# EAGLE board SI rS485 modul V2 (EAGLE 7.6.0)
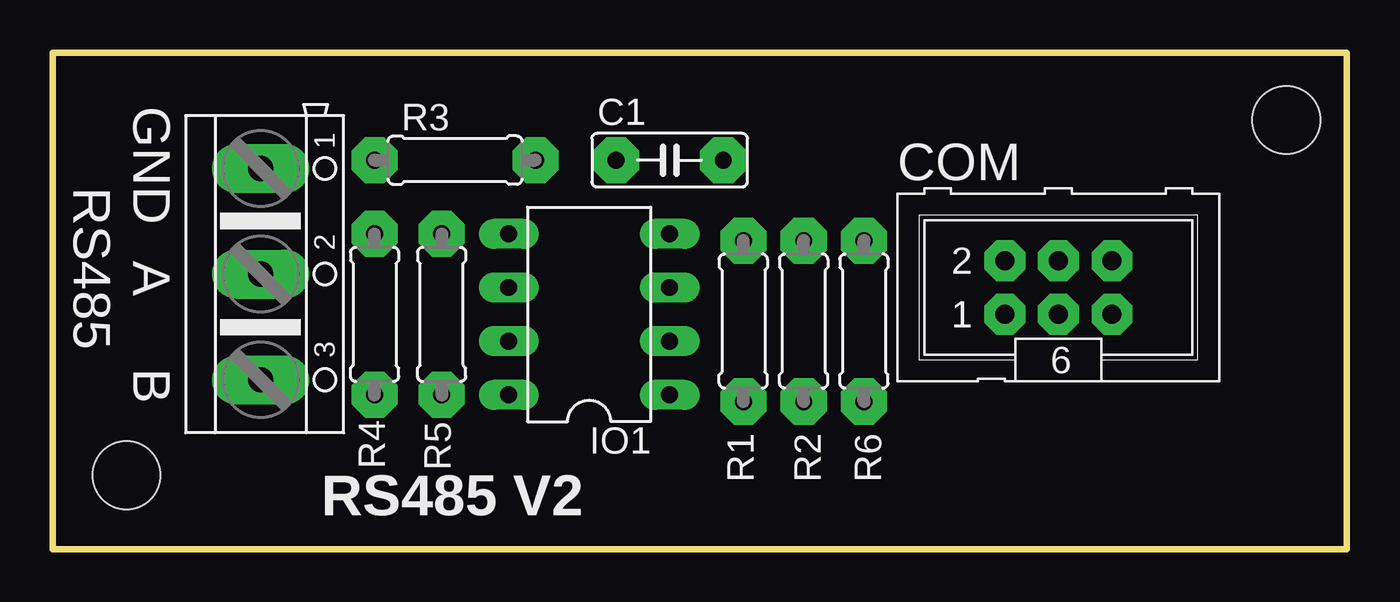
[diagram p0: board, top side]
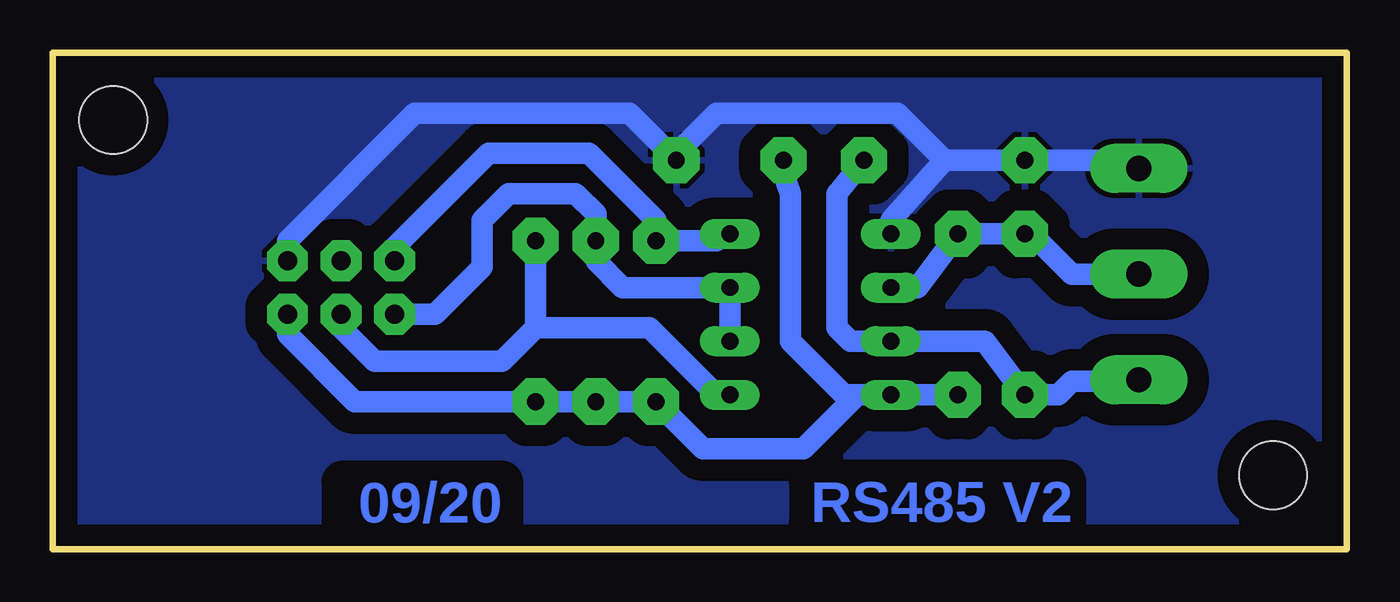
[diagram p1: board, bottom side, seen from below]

Size 61.28 x 23.5 mm. Coordinates in mm from the lower left corner, seen from the top.
Outline: 0,23.5 61.28,23.5 61.28,0 0,0 0,23.5
Copper layers (1*16): Top 0.035mm / dielectric 1.5mm / Bottom 0.035mm
Design rules "default": minimum track width 10mil, minimum drill 24mil, track to track 8mil, track to pad 8mil, pad to pad 8mil, via to via 8mil, smd to smd 8mil, copper to edge 40mil, drill to drill 8mil, minimum pad ring 10mil, minimum via ring 8mil, stop-mask expansion 4mil, vias tented up to drill 0mil, thermal gap 10mil
Holes 3.2 mm at 58.42,20.32 3.49,3.49

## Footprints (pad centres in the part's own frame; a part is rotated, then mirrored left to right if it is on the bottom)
C050-025X075 = drill 0.8 pad 2.184 octagon: 1 -2.54,0; 2 2.54,0
ML6 = drill 0.9 pad 1.93 octagon: 1 -2.54,-1.27; 2 -2.54,1.27; 3 0,-1.27; 4 0,1.27; 5 2.54,-1.27; 6 2.54,1.27
DIL08 = drill 0.8 pad 1.422 long: 1 -3.81,-3.81; 2 -1.27,-3.81; 3 1.27,-3.81; 4 3.81,-3.81; 5 3.81,3.81; 6 1.27,3.81; 7 -1.27,3.81; 8 -3.81,3.81
0207/7 = drill 0.8 pad 2.184 octagon: 1 -3.81,0; 2 3.81,0
AK500/3 = drill 1.2 pad 2.311 long: 1 -5.004,0; 2 0,0; 3 5.004,0

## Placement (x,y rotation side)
C1  100n  [C050-025X075]  29.21,18.41 0 top
COM  [ML6]  47.62,12.38 0 top
IO1  MAX485  [DIL08]  25.4,11.11 90 top
R1  10k  [0207/7]  32.7,10.79 90 top
R2  10k  [0207/7]  35.56,10.79 90 top
R3  20k  [0207/7]  19.05,18.41 0 top
R4  120  [0207/7]  15.24,11.11 90 top
R5  20k  [0207/7]  18.41,11.11 270 top
R6  10k  [0207/7]  38.42,10.79 90 top
RS485  [AK500/3]  9.84,13.02 270 top

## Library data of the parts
C1 COM IO1 R1-R6 RS485 = 11moje

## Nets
GND: C1.2 COM.6 IO1.5 R3.1 RS485.1
S$1: C1.1 COM.5 IO1.8 R1.1 R2.1 R5.2 R6.1
S$5: COM.1 IO1.2 IO1.3 R2.2
S$7: IO1.6 R4.2 R5.1 RS485.2
S$10: IO1.7 R3.2 R4.1 RS485.3
S$13: COM.3 IO1.1 R6.2
S$16: COM.2 IO1.4 R1.2

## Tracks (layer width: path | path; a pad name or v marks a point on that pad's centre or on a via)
GND
  Bottom 1.016: IO1.5 21.59,15.56 19.05,18.41 | 19.05,18.41 R3.1 10.48,18.41 10.08,18.02 RS485.1 | 19.05,18.41 21.27,20.64 29.84,20.64 32.07,18.41 C1.2 33.97,20.64 44.13,20.64 50.16,14.61 COM.6
  pour Bottom (isolate 1.016): 0,23.5 61.28,23.5 61.28,0 0,0
S$1
  Bottom 1.016: R5.2 IO1.8 23.18,7.3 | 23.18,7.3 23.81,7.3 26.35,9.84 26.35,16.83 26.67,17.78 C1.1 | R1.1 32.38,6.99 | R1.1 R2.1 R6.1 46.99,6.99 50.16,10.16 COM.5 | R1.1 30.48,4.76 25.72,4.76 23.18,7.3
S$5
  Bottom 1.016: IO1.2 IO1.3 34.29,12.38 35.56,13.65 R2.2 35.56,15.88 36.51,16.83 39.69,16.83 40.96,15.56 40.96,13.34 43.18,11.11 COM.1
S$7
  Bottom 1.016: IO1.6 20.32,12.38 R5.1 R4.2 14.92,14.92 13.02,13.02 RS485.2 9.53,13.02
S$10
  Bottom 1.016: R3.2 24.13,16.83 24.13,10.48 23.5,9.84 IO1.7 17.14,9.84 R4.1 13.65,7.3 13.02,7.94 9.84,7.94 RS485.3
S$13
  Bottom 1.016: 38.42,10.79 38.42,10.48 40.01,8.89 46.04,8.89 47.62,10.48 COM.3 | 38.42,10.79 R6.2 | IO1.1 29.84,7.3 33.02,10.48 38.1,10.48 38.42,10.79
S$16
  Bottom 1.016: IO1.4 29.53,14.92 29.84,14.61 R1.2 32.7,15.56 35.88,18.73 40.64,18.73 45.09,14.29 COM.2

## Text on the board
Bottom: 09/20 | RS485 V2
tNames: GND | A | B | RS485 V2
